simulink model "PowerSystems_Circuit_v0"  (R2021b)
settings: Solver=VariableStepAuto  StartTime=0.0  StopTime=60e-3  RelTol=1e-3
libraries: eeTransforms x1, spsThreePhaseSeriesRLCBranchLib x1, spsThreePhaseSeriesRLCLoadLib x1, spsThreePhaseVIMeasurementLib x1, spsThreePhaseSourceLib x1, spspowerguiLib x1

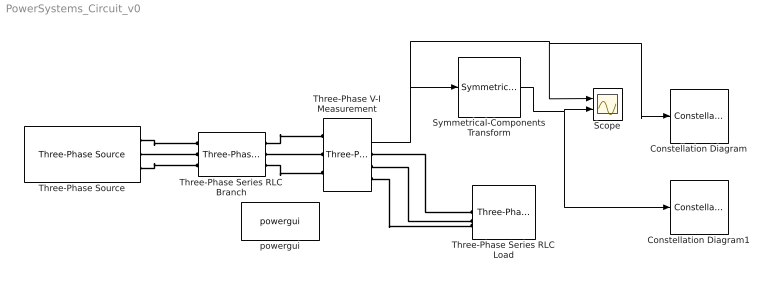
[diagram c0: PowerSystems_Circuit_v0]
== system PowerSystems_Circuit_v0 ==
  Constellation Diagram : ConstellationDiagram
  Constellation Diagram1 : ConstellationDiagram
  Scope : Scope  NumInputPorts=2
  Symmetrical-Components Transform : eeTransforms/Symmetrical-Components Transform  PowerInvariant=off
  Three-Phase Series RLC Branch : spsThreePhaseSeriesRLCBranchLib/Three-Phase Series RLC Branch  LConnTagsString=A|B|C  RConnTagsString=A|B|C  BranchType=R  Resistance=10  Inductance=0  Capacitance=0  Measurements=None
  Three-Phase Series RLC Load : spsThreePhaseSeriesRLCLoadLib/Three-Phase Series RLC Load  LConnTagsString=A|B|C  Configuration=Delta  NominalVoltage=380  Vabc=[1e3 1e3 1e3]  Vabcp=[1e3 1e3 1e3]  NominalFrequency=50  UnbalancedPower=on  ActivePower=10e3  InductivePower=100  CapacitivePower=100  Pabc=[1 1 1]*380  QLabc=[0 0 0]  QCabc=[0 0 0]  Pabcp=[1 1 2]*1e3  QLabcp=[100 90 110]*0  QCabcp=[100 90 110]*0  Measurements=None  LoadType=constant Z
  Three-Phase V-I Measurement : spsThreePhaseVIMeasurementLib/Three-Phase V-I Measurement  VoltageMeasurement=phase-to-ground  SetLabelV=off  LabelV=Vabc  Vpu=off  VpuLL=off  CurrentMeasurement=yes  SetLabelI=off  LabelI=Iabc  Ipu=off  Pbase=100e6  Vbase=500e3  OutputType=Complex  PhasorSimulation=on  PSBequivalent=0
  Three-Phase Source : spsThreePhaseSourceLib/Three-Phase Source  InternalConnection=Yg  VoltagePhases=off  Voltage=380  PhaseAngle=0  Voltage_phases=[25e3 25e3 25e3]/sqrt(3)  PhaseAngles_phases=[0 -120 +120]  Frequency=50  NonIdealSource=on  SpecifyImpedance=off  Resistance=0  Inductance=0  ShortCircuitLevel=100e6  BaseVoltage=380  XRratio=7  BusType=swing  Pref=10e3  Qref=0  Prefabc=[10e3, 10e3, 10e3]  Qrefabc=[0, 0, 0]  Qmin=-inf  Qmax=inf
  powergui : spspowerguiLib/powergui  Priority=1  SimulationMode=Discrete phasor  SampleTime=50e-6  frequency=50  Iterations=50  frequencyindice=50  Pbase=100e6  ErrMax=1e-4  UnitsV=kV  UnitsW=MW  buscounter=0  FunctionMessages=off  echomessages=off  EnableUseOfTLC=off  CurrentSourceSwitches=off  DisableSnubberDevices=off  DisableRonSwitches=off  DisableVfSwitches=off  DisplayEquations=off  AutomaticDiscreteSolvers=off  SolverType=Tustin/Backward Euler (TBE)  Interpol=off  ExternalGateDelay=off  methode=off  Ts=100  x0status=blocks  SPID=on  SwTol=0  HookPort=off  NonlinearTolerance=1e-4  nMaxIteration=100  ContinueOnMaxIteration=off  RestoreLinks=warning  ResistiveCurrentMeasurement=off  Frange=[0:2:500]  Ylog=off  Xlog=on  ShowGrid=off  save=off  variable=ZData  structure=0  ZoomFFT=off  StartTime=0.0  cycles=1  DisplayStyle=1  fundamental=60  FreqAxis=off  MaxFrequency=1000  frequencyindicesteady=1  RmsSteady=1  display=off
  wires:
  Symmetrical-Components Transform/1 -> Constellation Diagram1/1, Scope/2
  Three-Phase V-I Measurement/2 -> Constellation Diagram/1, Scope/1, Symmetrical-Components Transform/1
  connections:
  Three-Phase Source/RConn1 -- Three-Phase Series RLC Branch/LConn1
  Three-Phase Source/RConn2 -- Three-Phase Series RLC Branch/LConn2
  Three-Phase Source/RConn3 -- Three-Phase Series RLC Branch/LConn3
  Three-Phase Series RLC Branch/RConn1 -- Three-Phase V-I Measurement/LConn1
  Three-Phase Series RLC Branch/RConn2 -- Three-Phase V-I Measurement/LConn2
  Three-Phase Series RLC Branch/RConn3 -- Three-Phase V-I Measurement/LConn3
  Three-Phase V-I Measurement/RConn1 -- Three-Phase Series RLC Load/LConn1
  Three-Phase V-I Measurement/RConn2 -- Three-Phase Series RLC Load/LConn2
  Three-Phase V-I Measurement/RConn3 -- Three-Phase Series RLC Load/LConn3
